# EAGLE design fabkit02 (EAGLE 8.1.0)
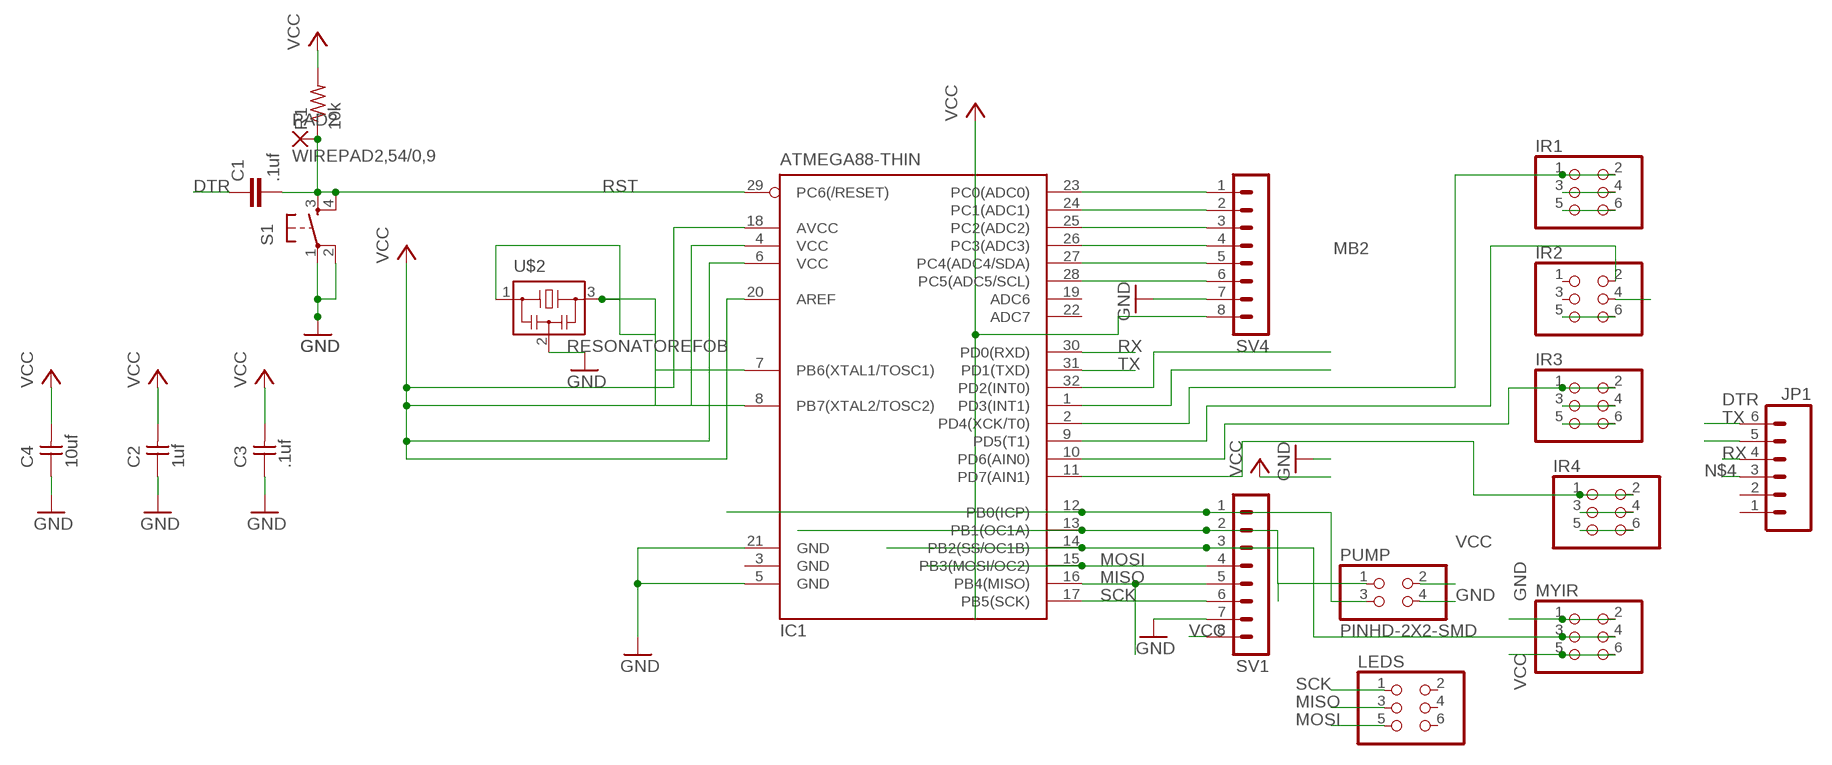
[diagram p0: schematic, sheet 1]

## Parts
C1  .1uf  C-EUC1206  [C1206]
C2  1uf  UNPOLARIZED_CAPACITOR1206  [1206]
C3  .1uf  UNPOLARIZED_CAPACITOR1206  [1206]
C4  10uf  UNPOLARIZED_CAPACITOR1206  [1206]
IC1  ATMEGA88-THIN  [TQFP32-08THIN]
IR1  PINHD-2X3-SMD  [2X03SMD]
IR2  PINHD-2X3-SMD  [2X03SMD]
IR3  PINHD-2X3-SMD  [2X03SMD]
IR4  PINHD-2X3-SMD  [2X03SMD]
JP1  M06SMD  [1X06-SMD]
LEDS  PINHD-2X3-SMD  [2X03SMD]
MYIR  PINHD-2X3-SMD  [2X03SMD]
PAD2  WIREPAD2,54/0,9  [2,54/0,9]
PUMP  PINHD-2X2-SMD  [2X02SMD]
R1  10k  RESISTOR1206  [1206]
S1  6MM_SWITCH6MM_SWITCH  [6MM_SWITCH]
SV1  MA08-1  [MA08-1]
SV4  MA08-1  [MA08-1]
U$2  RESONATOREFOB  [EFOBM]

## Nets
ADC0: IC1.23(PC0(ADC0)) SV4.1
ADC1: IC1.24(PC1(ADC1)) SV4.2
ADC2: IC1.25(PC2(ADC2)) SV4.3
ADC3: IC1.26(PC3(ADC3)) SV4.4
ADC4: IC1.27(PC4(ADC4/SDA)) SV4.5
ADC5: IC1.28(PC5(ADC5/SCL)) SV4.6
B1: IC1.12(PB0(ICP)) PUMP.3 SV1.1
B2: IC1.13(PB1(OC1A)) PUMP.1 SV1.2
DTR: C1.1 JP1.6
GND: C2.1 C3.1 C4.1 IC1.5(GND) IC1.21(GND) IR1.3 IR1.4 IR2.4 IR3.3 IR3.4 IR4.3 IR4.4 MYIR.1 MYIR.2 PUMP.4 S1.1(P) S1.2(P1) SV1.7 SV4.7 U$2.2
MA1: IC1.2(PD4(XCK/T0)) IR1.1 IR1.2
MA2: IC1.9(PD5(T1)) IR2.2
MB1: IC1.10(PD6(AIN0)) IR3.1 IR3.2
MB2: IC1.11(PD7(AIN1)) IR4.1 IR4.2
MISO: IC1.16(PB4(MISO)) LEDS.3 SV1.5
MOSI: IC1.15(PB3(MOSI/OC2)) LEDS.5 SV1.4
N$1: IC1.8(PB7(XTAL2/TOSC2)) U$2.1
N$4: JP1.3
N$5: IC1.32(PD2(INT0))
N$9: IC1.7(PB6(XTAL1/TOSC1)) U$2.3
N$18: IC1.14(PB2(SS/OC1B)) MYIR.3 MYIR.4 SV1.3
PD3: IC1.1(PD3(INT1))
RST: C1.2 IC1.29(PC6(/RESET)) PAD2.1(P) R1.1 S1.3(S) S1.4(S1)
RX: IC1.30(PD0(RXD)) JP1.4
SCK: IC1.17(PB5(SCK)) LEDS.1 SV1.6
TX: IC1.31(PD1(TXD)) JP1.5
VCC: C2.2 C3.2 C4.2 IC1.4(VCC) IC1.6(VCC) IC1.18(AVCC) IC1.20(AREF) IR1.5 IR1.6 IR2.5 IR2.6 IR3.5 IR3.6 IR4.5 IR4.6 MYIR.5 MYIR.6 PUMP.2 R1.2 SV1.8 SV4.8
Unconnected: IC1.19(ADC6) IC1.22(ADC7) IR2.1 IR2.3 JP1.1 JP1.2 LEDS.2 LEDS.4 LEDS.6

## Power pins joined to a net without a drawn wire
GND: IC1.3(GND)

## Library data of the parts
C1 = rcl:C-EU: CAPACITOR, European symbol
C2-C4 = ng:UNPOLARIZED_CAPACITOR: unpolarized_capacitor
IC1 = fab:ATMEGA88-THIN
IR1-IR4 LEDS MYIR = fab:PINHD-2X3-SMD: PIN HEADER
JP1 = SparkFun:M06: Header 6 Standard 6-pin 0.1" header. Use with straight break away headers (SKU : PRT-00116), right angle break away headers (PRT-00553), swiss pins (PRT-00743), machine pins (PRT-00117), and female headers (PRT-00115). Molex polarized connector foot print use with SKU : PRT-08094 with associated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
PAD2 = wirepad:WIREPAD: Wire PAD connect wire on PCB
PUMP = fab:PINHD-2X2-SMD
R1 = ng:RESISTOR
S1 = ng:6MM_SWITCH: OMRON SWITCH
SV1 SV4 = con-lstb:MA08-1: PIN HEADER
U$2 = fab:RESONATOR

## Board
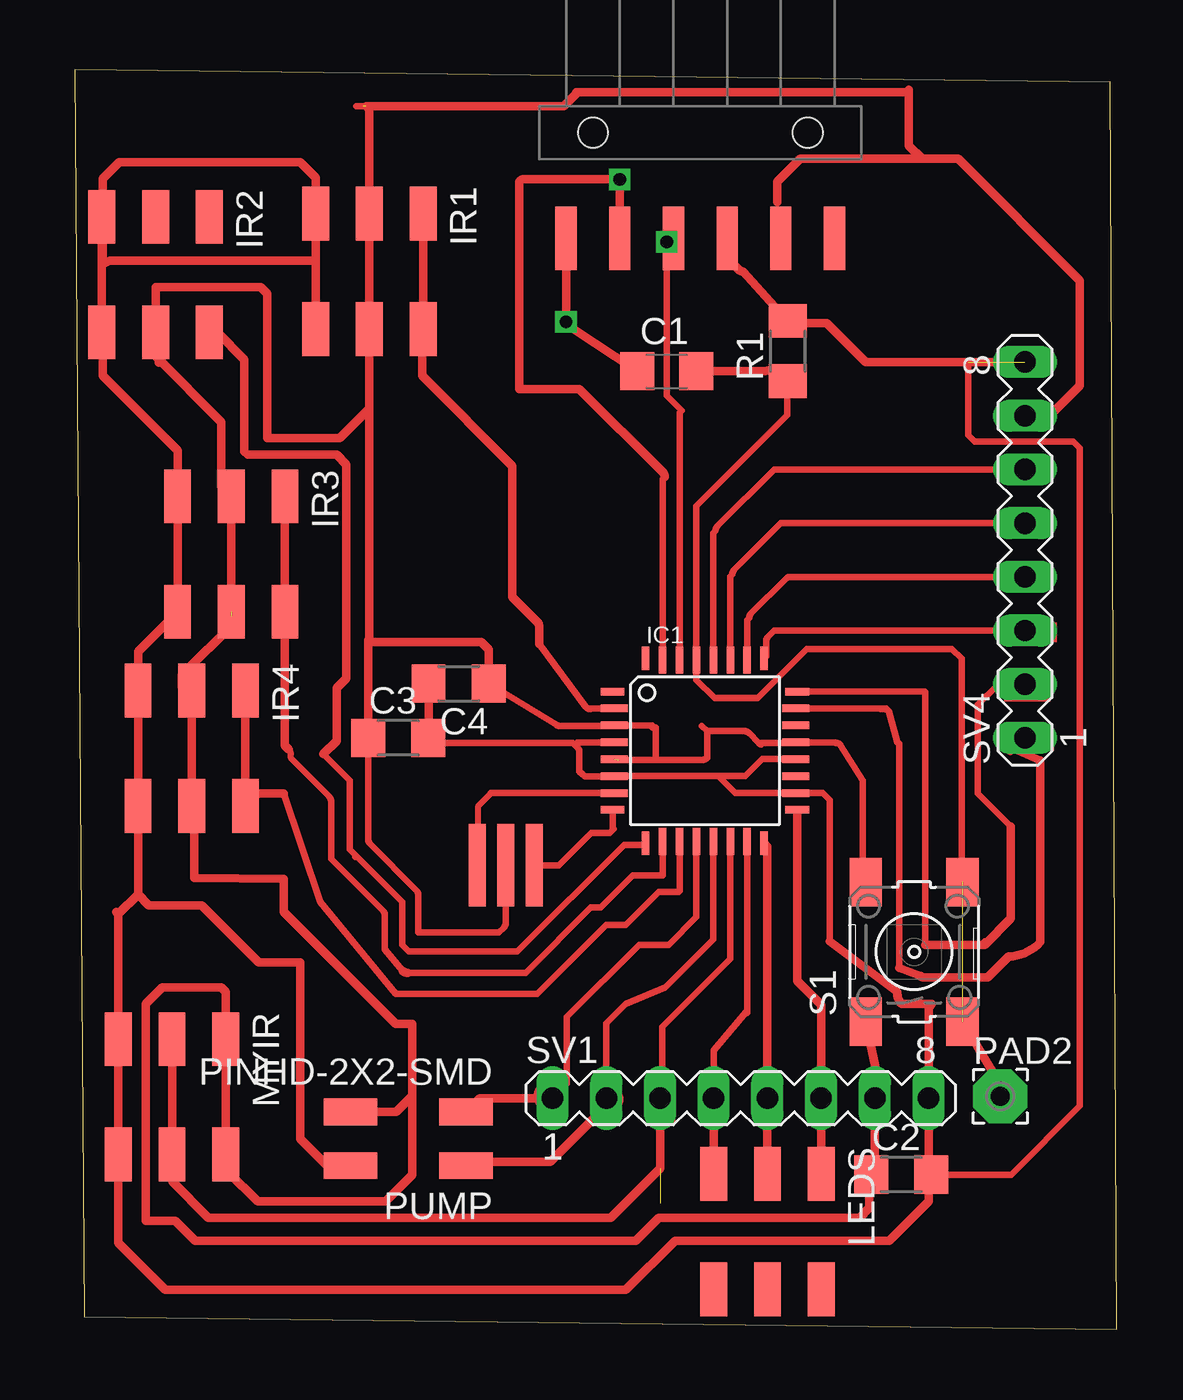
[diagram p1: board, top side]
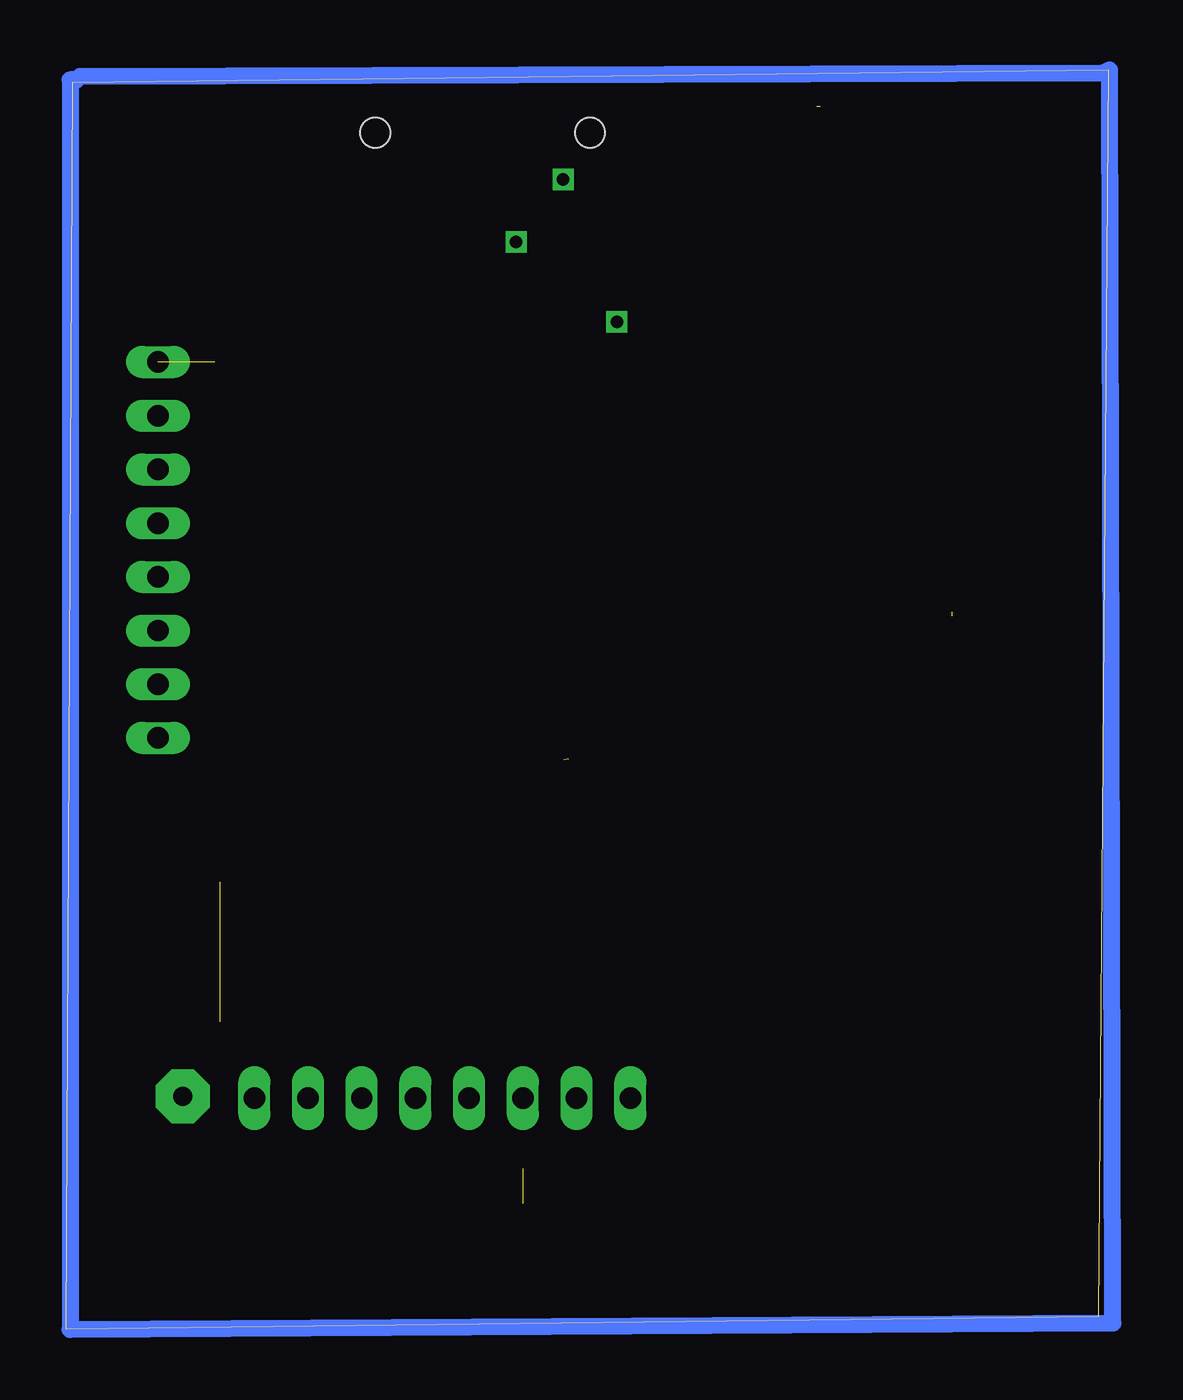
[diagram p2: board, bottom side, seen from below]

Size 49.29 x 59.59 mm. Coordinates in mm from the lower left corner, seen from the top.
Outline: 0.47,0.6 49.29,0 48.98,59 0,59.6 0.47,0.6
Copper layers (1*16): Top 0.035mm / dielectric 1.5mm / Bottom 0.035mm
Design rules "default": minimum track width 10mil, minimum drill 24mil, track to track 8mil, track to pad 8mil, pad to pad 8mil, via to via 8mil, smd to smd 8mil, copper to edge 40mil, drill to drill 8mil, minimum pad ring 10mil, minimum via ring 8mil, stop-mask expansion 4mil, vias tented up to drill 0mil, thermal gap 10mil

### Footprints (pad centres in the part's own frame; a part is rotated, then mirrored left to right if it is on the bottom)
C1206 = smd 1.6 x 1.8: 1 -1.4,0; 2 1.4,0
1206 = smd 1.6 x 1.803: 1 -1.422,0; 2 1.422,0
TQFP32-08THIN = smd 1.118 x 0.356: 1 -4.369,2.8; 8 -4.369,-2.8; 17 4.369,-2.8; 24 4.369,2.8 | smd 1.27 x 0.356: 2 -4.293,2; 3 -4.293,1.2; 4 -4.293,0.4; 5 -4.293,-0.4; 6 -4.293,-1.2; 7 -4.293,-2; 18 4.293,-2; 19 4.293,-1.2; 20 4.293,-0.4; 21 4.293,0.4; 22 4.293,1.2; 23 4.293,2 | smd 0.356 x 1.118: 9 -2.8,-4.369; 16 2.8,-4.369; 25 2.8,4.369; 32 -2.8,4.369 | smd 0.356 x 1.27: 10 -2,-4.293; 14 1.2,-4.293; 15 2,-4.293; 26 2,4.293; 27 1.2,4.293; 31 -2,4.293 | smd 0.35 x 1.27: 11 -1.2,-4.293; 12 -0.4,-4.293; 13 0.4,-4.293; 28 0.4,4.293; 29 -0.4,4.293; 30 -1.2,4.293
2X03SMD = smd 2.54 x 1.27: 1 -2.54,2.54; 2 2.92,2.54; 3 -2.54,0; 4 2.92,0; 5 -2.54,-2.54; 6 2.92,-2.54
1X06-SMD = smd 1 x 3: 1 -6.35,5; 2 -3.81,5; 3 -1.27,5; 4 1.27,5; 5 3.81,5; 6 6.35,5 | hole 1.4: -5.08,0; 5.08,0
2,54/0,9 = drill 0.914 pad 2.54 octagon: 1 0,0
2X02SMD = smd 2.54 x 1.27: 1 -2.54,1.27; 2 2.92,1.27; 3 -2.54,-1.27; 4 2.92,-1.27
6MM_SWITCH = smd 2.286 x 1.524: 1 -3.302,2.286; 2 3.302,2.286; 3 -3.302,-2.286; 4 3.302,-2.286
MA08-1 = drill 1.016 long: 1 -8.89,0; 2 -6.35,0; 3 -3.81,0; 4 -1.27,0; 5 1.27,0; 6 3.81,0; 7 6.35,0; 8 8.89,0
EFOBM = smd 0.8 x 3.9: 1 -1.35,0; 2 0,0; 3 1.35,0

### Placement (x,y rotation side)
C1  28.01,45.33 0 top
C2  39.1,7.33 0 top
C3  15.31,27.99 0 top
C4  18.16,30.55 180 top
IC1  29.81,27.38 0 top
IR1  13.94,50.25 270 top
IR2  3.83,50.1 270 top
IR3  7.41,36.87 270 top
IR4  5.54,27.69 270 top
JP1  29.59,56.62 180 top
LEDS  32.77,4.82 270 top
MYIR  4.61,11.2 270 top
PAD2  43.78,11.03 0 top
PUMP  15.97,9.02 180 top
R1  33.72,46.29 90 top
S1  39.71,17.87 90 top
SV1  31.5,10.94 0 top
SV4  44.95,36.88 90 top
U$2  20.39,21.96 180 top

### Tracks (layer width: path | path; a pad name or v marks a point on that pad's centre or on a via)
ADC0
  Top 0.305: 38.99,17.11 38.99,27.72 arc45 38.9,27.79 38.51,29.26 | 38.51,29.26 arc45 38.13,29.35 | IC1.23 38.39,29.38 38.51,29.26
  Top 0.406: SV4.1 44.24,27.37 arc45 44.17,27.58 45.68,26.91 45.68,18.33 arc-45 44.19,17.64 43.19,16.65 40.21,16.65 arc-45 39.99,16.74 38.99,17.11
ADC1
  Top 0.305: 43.04,18.2 43.04,18.36 | 40.24,18.2 40.24,30.15 40.21,30.18 IC1.24 | 44.28,23.8 42.73,25.36 42.73,29.56 43.66,30.49 44.91,30.49 SV4.2
  Top 0.406: 40.24,18.2 43.04,18.2 44.28,19.45 44.28,23.8
ADC2
  Top 0.305: SV4.3 33.09,33.07 32.8,32.79 arc45 32.71,32.56 32.71,31.85 IC1.25
ADC3
  Top 0.305: SV4.4 33.85,35.61 arc45 33.63,35.52 32,33.89 arc45 31.91,33.67 31.81,33.57 IC1.26
ADC4
  Top 0.305: SV4.5 33.4,38.15 31.2,35.95 arc45 31.11,35.72 31.01,35.63 IC1.27
ADC5
  Top 0.305: SV4.6 33.09,40.69 30.4,38.01 arc45 30.31,37.78 30.21,37.68 IC1.28
B1
  Top 0.305: SV1.1 23.28,11.61 23.28,14.78 26.7,18.2 28.1,18.2 29.41,19.51 IC1.12
  Top 0.406: 22.7,10.94 arc45 22.61,10.71 SV1.1 19.16,10.94 PUMP.3
B2
  Top 0.305: SV1.2 25.15,14.47 26.08,15.4 27.95,16.18 30.21,18.45 IC1.13
  Top 0.406: 25.24,11.57 arc45 25.15,11.35 SV1.2 25.15,10.58 22.5,7.93 18.69,7.93 PUMP.1
DTR  (via drill 0.6)
  Top 0.406: C1.1 23.56,47.36 arc-90 v23.24,47.67 JP1.6
GND  (3 unrouted)
  Top 0.305: C4.1 22.74,28.65 arc45 22.96,28.55 25.52,28.55 IC1.3 27.32,28.58 27.32,28.47 27.48,28.47 27.48,26.95 | 27.48,26.95 25.75,26.95 | 27.48,26.95 29.71,26.95 arc45 29.91,27.04 29.91,28.31 | U$2.2 20.39,19.23 arc-45 20.29,19.01 20.07,18.78 16.26,18.78 16.26,20.55 arc45 16.17,20.78 13.98,22.97 arc-45 13.88,23.19 C3.1 | 29.91,28.31 31.69,28.31 arc-45 31.91,28.21 32.37,27.76 | 32.37,27.76 32.45,27.67 arc-45 32.65,27.75 | 37.28,20.42 37.28,25.98 36.22,27.66 arc45 36,27.75 35.97,27.78 IC1.21 34.11,27.76 32.37,27.76 | 29.66,28.55 29.91,28.31 | 13.32,57.87 13.63,57.87 | 23.74,58.49 24.16,58.49 24.21,58.54
  Top 0.406: S1.1 37.94,12.13 arc45 37.85,11.9 SV1.7 37.85,7.5 C2.1 37.59,7.24 37.59,5.76 37.13,5.29 27.64,5.29 26.55,4.2 5.7,4.2 4.77,5.13 3.37,5.13 3.37,15.4 4.14,16.18 6.94,16.18 7.15,15.97 MYIR.1 MYIR.2 7.26,8.18 7.26,7.47 8.66,6.07 14.72,6.07 15.97,7.31 15.97,11.05 | 37.28,20.42 arc-45 S1.2 | SV4.7 46.13,43.23 47.55,44.65 47.55,49.63 41.79,55.39 40.08,55.39 | 40.08,55.39 34.33,55.39 33.24,54.3 33.24,53.34 | 40.08,55.39 39.46,56.01 39.46,58.65 39.35,58.54 24.21,58.54 23.72,58.54 | 13.88,29.31 C3.1 13.88,32.61 13.94,32.67 | C4.1 19.59,32.16 19.23,32.52 14.1,32.52 13.94,32.67 | 23.74,58.49 23.13,57.87 13.79,57.87 13.94,57.72 IR1.3 IR1.4 13.94,43.56 | 13.94,43.56 12.54,42.16 9.12,42.16 9.12,49.01 8.81,49.32 3.83,49.32 3.83,47.76 | 3.83,47.76 IR2.4 3.83,46.05 6.94,42.94 6.94,39.88 IR3.3 7.41,33.76 7.72,33.45 7.57,33.45 5.08,30.96 5.08,30.39 IR4.3 IR4.4 | 3.99,45.74 3.99,47.61 3.83,47.76 | PUMP.4 15.21,10.29 15.97,11.05 | 15.97,11.05 15.97,14.47 15.19,14.47 9.9,19.76 9.9,21.31 5.66,21.35 5.66,24.66 IR4.4 | 13.94,32.67 13.94,43.56 | 5.86,24.46 IR4.4
MA1
  Top 0.305: 21.97,32.43 24.18,29.45 arc45 24.41,29.35 24.41,29.38 IC1.2
  Top 0.406: 21.97,32.43 21.97,33.25 arc45 21.88,33.48 20.7,34.66 20.7,40.85 16.43,45.12 16.43,47.87 16.48,47.92 | 16.48,47.92 IR1.2 | 16.48,47.92 IR1.1
MA2
  Top 0.292: 11.77,27.23 13.01,25.98
  Top 0.305: 13.01,25.98 13.01,22.71 13.28,22.45 13.28,22.36 13.37,22.36 15.5,20.23 15.5,18.2 15.81,17.89 20.95,17.89 25.99,22.93 26.93,22.93 IC1.9
  Top 0.406: IR2.2 6.75,47.18 8.03,45.89 8.03,41.54 8.19,41.38 12.39,41.38 12.86,40.92 12.86,30.8 12.39,30.34 12.39,27.85 11.77,27.23
MB1
  Top 0.292: 12.04,25.22 10.23,27.04 10.23,27.22 arc45 10.13,27.45
  Top 0.305: 15.76,16.88 21.34,16.88 24.42,19.96 24.88,19.96 26.39,21.47 27.81,21.47 IC1.10 | 15.53,16.97 14.67,17.98 14.67,19.6 arc45 14.58,19.83 12.13,22.27 12.13,25 arc45 12.04,25.22
  Top 0.406: 15.76,16.88 arc-45 15.53,16.97 | IR3.1 IR3.2 | 10.13,27.45 9.95,27.63 IR3.2 | IR3.2 10.06,33.85
MB2
  Top 0.305: 9.9,25.36 11.61,20.23 15.19,15.87 21.88,15.87 25.15,19.14 26.08,19.14 27.64,20.69 28.57,20.69 28.61,20.74 IC1.11
  Top 0.406: IR4.1 IR4.2 8.67,25.36 9.9,25.36
MISO
  Top 0.305: 32.71,11 SV1.5
  Top 0.406: 32.77,9.65 SV1.5 | SV1.5 LEDS.3 | SV1.5 32.77,22.86 IC1.16
MOSI
  Top 0.305: SV1.4 30.23,13.2 31.76,15.04 31.81,14.98 IC1.15
  Top 0.406: SV1.4 LEDS.5
N$1
  Top 0.305: 21.72,23.51 U$2.1 22.89,21.96 24.43,23.49 25.3,23.49 25.49,23.68 25.44,23.68 IC1.8
  Top 0.406: 21.94,23.6 arc-45 21.72,23.51
N$3
  Bottom 0.813: 0.25,59.43 48.64,59.27 48.79,59.12 49.1,59.12 49.1,0 -0.21,0.31 -0.06,59.59 0.25,59.43
N$9
  Top 0.292: 19.7,25.35 19.08,24.74 19.08,22 U$2.3
  Top 0.305: IC1.7 19.7,25.38 19.7,25.35
  Top 0.406: U$2.3 arc45 19.12,22.15
N$18  (1 unrouted)
  Top 0.305: IC1.14 31.01,17.54 27.79,14.31 27.79,11.04 SV1.3
  Top 0.406: SV1.3 27.69,11.98 arc-45 27.78,12.21 | SV1.3 27.69,7.62 25.36,5.29 6.32,5.29 4.61,7 MYIR.4 MYIR.3 | SV1.3 27.69,12.11
RST  (1 unrouted)
  Top 0.305: 33.7,44.85 33.7,43.25 29.41,38.96 IC1.29 29.41,30.74 30.28,29.87 32.3,29.87 34.64,32.2 41.48,32.2 41.95,31.74 41.95,21.22 S1.4
  Top 0.406: C1.2 32.66,45.33 arc-45 33.51,45.24 R1.1 33.7,44.85 | PAD2.1 43.47,12.03 arc45 43.37,12.25 S1.3
RX  (via drill 0.6)
  Top 0.305: v28.01,51.46 28.01,44.18 28.71,43.48 28.61,43.38 IC1.30
  Top 0.406: JP1.4 arc90 v28.01,51.46
SCK
  Top 0.406: 35.31,9.44 SV1.6 | SV1.6 LEDS.1 | SV1.6 35.31,15.35 34.17,16.49 34.17,24.57 IC1.17
TX  (via drill 0.6)
  Top 0.305: IC1.31 27.81,40.24 27.91,40.33
  Top 0.406: JP1.5 v25.78,54.41 21.34,54.41 arc90 21.02,54.25 21.02,44.5 23.88,44.5 27.82,40.56 arc-45 27.91,40.33
VCC  (1 unrouted)
  Top 0.305: 17.1,27.75 23.56,27.75 23.79,27.53 | 23.79,27.53 arc-45 23.88,27.3 23.88,26.4 24.03,26.25 arc45 24.26,26.15 25.52,26.15 IC1.6 30.44,26.18 | 35.73,18.36 35.73,25.05 35.39,25.38 IC1.18 31.24,25.38 30.44,26.18 | IC1.4 23.79,27.78 23.79,27.53 | 30.44,26.18 31.73,26.18 32.53,26.98 IC1.20 | 42.26,45.77 42.26,42.32 42.57,42.01 47.24,42.01 47.55,41.69 47.55,10.58 44.3,7.33 C2.2
  Top 0.406: 30.86,50.68 31.41,50.14 arc45 31.63,50.05 R1.2 33.83,47.61 35.57,47.61 37.41,45.77 SV4.8 | C4.2 16.74,28.02 arc-45 C3.2 16.87,27.85 arc45 17.1,27.75 | 35.73,18.36 38.9,15.96 arc45 39.12,15.4 40.55,15.4 40.48,15.34 arc45 40.39,15.11 SV1.8 40.39,7.93 | 11.4,50.56 IR1.5 11.4,54.5 10.68,55.23 2.12,55.23 1.34,54.45 1.34,52.58 | 11.4,50.56 IR1.6 | 11.4,50.56 1.65,50.56 1.34,50.41 1.34,52.58 | 1.34,52.58 IR2.5 IR2.6 1.34,47.12 1.34,45.12 4.87,41.59 IR3.5 IR3.6 3,32.08 IR4.5 IR4.6 3,20.59 | PUMP.2 11.95,7.75 10.68,9.02 10.68,17.38 8.7,17.38 6.01,20.07 3.52,20.07 3,20.59 | 2.07,19.65 MYIR.5 MYIR.6 2.07,4.1 4.3,1.87 26.08,1.87 28.41,4.2 38.53,4.2 40.39,6.07 40.39,7.93 | 2.07,19.65 1.97,19.76 | 40.39,7.93 40.39,7.46 C2.2 | 3,20.59 2.07,19.65
(copper drawn outside any net)
  shapes: Top area x17, Top circle x2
